[IBIS Ver]   3.2
[File Name]   sprm296a.ibs
[File Rev]   1.0
[Date]   November 3, 2003
[Source]   File originated at Texas Instruments
[Copyright]   (c) 2003, Texas Instruments Inc.
[Component]   f2810pbk
[Manufacturer] Texas Instruments
[Package]
| Variable   Typ   Min   Max
R_pkg   0.063   0.061   0.064
L_pkg   2.512e-09   2.373e-10   2.8e-09
C_pkg   0.455e-13   0.4e-13   0.557e-13
[Pin] signal_name   model_name   R_pin   L_pin   C_pin
1   VDDAIO   NC   0.062 2.856e-09 0.429e-13
2   ADCINB0   ioh125   0.062 2.768e-09 0.518e-13
3   ADCINB1   ioh125   0.061 2.741e-09 0.555e-13
4   ADCINB2   ioh125   0.062 2.718e-09 0.542e-13
5   ADCINB3   ioh125   0.061 2.661e-09 0.499e-13
6   ADCINB4   ioh125   0.061 2.656e-09 0.526e-13
7   ADCINB5   ioh125   0.061 2.604e-09 0.498e-13
8   ADCINB6   ioh125   0.060 2.557e-09 0.432e-13
9   ADCINB7   ioh125   0.061 2.536e-09 0.437e-13
10   ADCREFM   ioh125   0.063 2.528e-09 0.411e-13
11   ADCREFP   ioh125   0.063 2.503e-09 0.376e-13
12   AVSSREFBG   ioh125   0.063 2.456e-09 0.366e-13
13   AVDDREFBG   ioh125   0.064 2.457e-09 0.374e-13
14   VDDA1   NC   0.065 2.457e-09 0.365e-13
15   VSSA1   NC   0.065 2.384e-09 0.330e-13
16   ADCRESEXT   ioh125   0.065 2.337e-09 0.356e-13
17   VSS   NC   0.065 2.341e-09 0.356e-13
18   MDRA   idg095_ouo435_ps1005   0.065 2.380e-09 0.329e-13
19   MDXA   idg095_ouo435   0.065 2.466e-09 0.366e-13
20   VDD   NC   0.065 2.481e-09 0.376e-13
21   MCLKRA   idg095_ouo435_ps1005   0.064 2.479e-09 0.368e-13
22   MFSXA   idg095_ouo435_ps1005   0.063 2.500e-09 0.376e-13
23   MCLKXA   idg095_ouo435_ps1005   0.063 2.528e-09 0.412e-13
24   MFSRA   idg095_ouo435_ps1005   0.062 2.551e-09 0.439e-13
25   VDDIO   NC   0.062 2.591e-09 0.435e-13
26   VSS   NC   0.062 2.636e-09 0.502e-13
27   SPICLKA   idg095_ouo435   0.062 2.663e-09 0.526e-13
28   SPISTEA   idg095_ouo435   0.062 2.676e-09 0.500e-13
29   VDD   NC   0.062 2.731e-09 0.543e-13
30   VSS   NC   0.062 2.763e-09 0.557e-13
31   SPISIMOA   idg095_ouo435   0.063 2.792e-09 0.520e-13
32   SPISOMIA   idg095_ouo435   0.064 2.889e-09 0.432e-13
33   PWM7   sw0145_ouo435_ups285   0.062 2.856e-09 0.429e-13
34   PWM8   sw0145_ouo435_ups285   0.062 2.768e-09 0.518e-13
35   PWM9   sw0145_ouo435_ups285   0.061 2.741e-09 0.555e-13
36   PWM10   sw0145_ouo435_ups285   0.062 2.718e-09 0.542e-13
37   PWM11   sw0145_ouo435_ups285   0.061 2.661e-09 0.499e-13
38   PWM12   sw0145_ouo435_ups285   0.061 2.656e-09 0.526e-13
39   VSS   NC   0.061 2.604e-09 0.498e-13
40   T3PWM_T3CMP   sw0145_ouo435_ups285   0.060 2.557e-09 0.432e-13
41   T4PWM_T4CMP   sw0145_ouo435_ups285   0.061 2.536e-09 0.437e-13
42   VDD   NC   0.063 2.528e-09 0.411e-13
43   CAP4_QEP3   sw0145_ouo435_ups285   0.063 2.503e-09 0.376e-13
44   CAP5_QEP4   sw0145_ouo435_ups285   0.063 2.456e-09 0.366e-13
45   CAP6_QEPI2   sw0145_ouo435_ups285   0.064 2.457e-09 0.374e-13
46   C4TRIPn   sw0145_ouo435_ups285   0.065 2.457e-09 0.365e-13
47   C5TRIPn   sw0145_ouo435_ups285   0.065 2.384e-09 0.330e-13
48   C6TRIPn   sw0145_ouo435_ups285   0.065 2.337e-09 0.356e-13
49   VDDIO   NC   0.065 2.341e-09 0.356e-13
50   TEST2   iog195   0.065 2.380e-09 0.329e-13
51   TEST1   iog195   0.065 2.466e-09 0.366e-13
52   VDD3VFL   NC   0.065 2.481e-09 0.376e-13
53   VSS   NC   0.064 2.479e-09 0.368e-13
54   TDIRB   sw0145_ouo435_ups285   0.063 2.500e-09 0.376e-13
55   TCLKINB   sw0145_ouo435_ups285   0.063 2.528e-09 0.412e-13
56   VDD   NC   0.062 2.551e-09 0.439e-13
57   X2   NC   0.062 2.591e-09 0.435e-13
58   X1/XCLKIN   NC   0.062 2.636e-09 0.502e-13
59   VSS   NC   0.062 2.663e-09 0.526e-13
60   T3CTRIP_PDPINTBn idg095_ouo435_ps1005   0.062 2.676e-09 0.500e-13
61   T4CTRIPn/EVBSOCn idg095_ouo435_ps1005   0.062 2.731e-09 0.543e-13
62   VSS   NC   0.062 2.763e-09 0.557e-13
63   VDD   NC   0.063 2.792e-09 0.520e-13
64	  CANTXA   idg095_ouo435_ps1005 		0.064 2.889e-09 0.43205e-
65	  CANRXA   idg095_ouo435_ps1005 		0.062 2.856e-09 0.42905e-
66	  SCITXDB	  idg095_ouo435   0.062 2.768e-09 0.518e-13
67	  SCIRXDB	  idg095_ouo435   0.061 2.741e-09 0.555e-13
68 	 PWM1	  idg095_ouo435_ps1005   0.062 2.718e-09 0.542e-13
69 	 PWM2   idg095_ouo435_ps1005   0.061 2.661e-09 0.499e-13
70 	 PWM3   idg095_ouo435_ps1005   0.061 2.656e-09 0.526e-13
71	  PWM4   idg095_ouo435_ps1005   0.061 2.604e-09 0.498e-13
72	  PWM5   idg095_ouo435_ps1005   0.060 2.557e-09 0.432e-13
73	  VSS   NC   0.061 2.536e-09 0.437e-13
74	  VDD   NC   0.063 2.528e-09 0.411e-13
75	  PWM6   idg095_ouo435_ps1005   0.063 2.503e-09 0.376e-13
76	 T1PWM_T1CMP	  idg095_ouo435_ps1005   0.063 2.456e-09 0.366e-13
77	  T2PWM_T2CMP	  idg095_ouo435_ps1005   0.064 2.457e-09 0.374e-13
78	 CAP1_QEP1	  idg095_ouo435_ps1005   0.065 2.457e-09 0.365e-13
79	 CAP2_QEP2	  idg095_ouo435_ps1005   0.065 2.384e-09 0.330e-13
80	 CAP3_QEPI1	  idg095_ouo435_ps1005   0.065 2.337e-09 0.356e-13
81	 T1CTRIP_PDPINTAn idg095_ouo435_ps1005   0.065 2.341e-09 0.356e-13
82	 VDD   NC   0.065 2.380e-09 0.329e-13
83 	VDDIO   NC   0.065 2.466e-09 0.366e-13
84	 T2CTRIPn/EVASOCn idg095_ouo435_ps1005   0.065 2.481e-09 0.376e-13
85	 TDIRA   idg095_ouo435_ps1005   0.064 2.479e-09 0.368e-13
86	 TCLKINA	  idg095_ouo435_ps1005   0.063 2.500e-09 0.376e-13
87	 XCLKOUT	  oui835   0.063 2.528e-09 0.412e-13
88	 VSS   NC   0.062 2.551e-09 0.439e-13
89	 C1TRIPn	  idg095_ouo435_ps1005   0.062 2.591e-09 0.435e-13
90	 C2TRIPn	  idg095_ouo435_ps1005   0.062 2.636e-09 0.502e-13
91	 C3TRIPn	  idg095_ouo435_ps1005   0.062 2.663e-09 0.526e-13
92	 TMS   idg095_ps1005   0.062 2.676e-09 0.500e-13
93	 TDO   oui835   0.062 2.731e-09 0.543e-13
94	 VDD   NC   0.062 2.763e-09 0.557e-13
95	 VSS   NC   0.063 2.792e-09 0.520e-13
96	 TDI   idg095_ps1005   0.064 2.889e-09 0.432e-13
97	 TESTSEL	  idg095_pe1005   0.062 2.856e-09 0.429e-13
98	 TRSTn   idg095_pe1005   0.062 2.768e-09 0.518e-13
99	 TCK   idg095_ps1005   0.061 2.741e-09 0.555e-13
100	 EMU0   idg095_oui835_ps1005   0.062 2.718e-09 0.542e-13
101	 XF_XPLLDIS	  idg095_oui835_ps1005   0.061 2.661e-09 0.499e-13
102	 VDD   NC   0.061 2.656e-09 0.526e-13
103	 VSS   NC   0.061 2.604e-09 0.498e-13
104   VDDIO   NC   0.060 2.557e-09 0.432e-13
105   EMU1   idg095_oui835_ps1005 		0.061 2.536e-09 0.437e-13
106   XINT1_XBIOn   idg095_ouo435   0.063 2.528e-09 0.411e-13
107   XNMI_XINT13   idg095_ouo435_ps1005 		0.063 2.503e-09 0.376e-13
108   XINT2_ADCSOC   idg095_ouo435   0.063 2.456e-09 0.366e-13
109   VSS   NC   0.064 2.457e-09 0.374e-13
110   VDD   NC   0.065 2.457e-09 0.365e-13
111   SCITXDA   idg095_ouo435_ps1005 		0.065 2.384e-09 0.330e-13
112   SCIRXDA   idg095_ouo435_ps1005 		0.065 2.337e-09 0.356e-13
113   XRSn   idg095_oum425_ps1005   0.065 2.341e-09 0.356e-13
114   VDD1   NC   0.065 2.380e-09 0.329e-13
115	  VSS1   NC   0.065 2.466e-09 0.366e-13
116   ADCBGREFIN   ioh125   0.065 2.481e-09 0.376e-13
117   VSSA2   NC   0.064 2.479e-09 0.368e-13
118   VDDA2   NC   0.063 2.500e-09 0.376e-13
119   ADCINA7   ioh125   0.063 2.528e-09 0.412e-13
120   ADCINA6   ioh125   0.062 2.551e-09 0.439e-13
121   ADCINA5   ioh125   0.062 2.591e-09 0.435e-13
122   ADCINA4   ioh125   0.062 2.636e-09 0.502e-13
123   ADCINA3   ioh125   0.062 2.663e-09 0.526e-13
124   ADCINA2   ioh125   0.062 2.676e-09 0.500e-13
125   ADCINA1   ioh125   0.062 2.731e-09 0.543e-13
126   ADCINA0   ioh125   0.062 2.763e-09 0.557e-13
127   ADCLO   ioh125   0.063 2.792e-09 0.520e-13
128   VSSAIO   NC   0.064 2.889e-09 0.432e-13
| End of package information
| Component idg095
[Component]   idg095
[Manufacturer]   Texas Instruments
[Package]
|   typ   min   max
R_pkg   0   0   0
L_pkg   0   0   0
C_pkg   0   0   0
[Pin]   signal_name   model_name   R_pin   L_pin   C_pin
   1   A   idg095   0   0   0
| Component idg095_oui835_ps1005
[Component]   idg095_oui835_ps1005
[Manufacturer]   Texas Instruments
[Package]
|   typ   min   max
R_pkg   0   0   0
L_pkg   0   0   0
C_pkg   0   0   0
[Pin]   signal_name   model_name   R_pin   L_pin   C_pin
   1   Y  idg095_oui835_ps1005   0   0   0
| Component idg095_oum425_ps1005
[Component]   idg095_oum425_ps1005
[Manufacturer]   Texas Instruments
[Package]
|   typ   min   max
R_pkg   0   0   0
L_pkg   0   0   0
C_pkg   0   0   0
[Pin]   signal_name   model_name   R_pin   L_pin   C_pin
   1   Y  idg095_oum425_ps1005   0   0   0
| Component idg095_ouo435_ps1005
[Component]   idg095_ouo435_ps1005
[Manufacturer]   Texas Instruments
[Package]
|   typ   min   max
R_pkg   0   0   0
L_pkg   0   0   0
C_pkg   0   0   0
[Pin]   signal_name   model_name   R_pin   L_pin   C_pin
   1   Y  idg095_ouo435_ps1005   0   0   0
| Component idg095_pe1005
[Component]   idg095_pe1005
[Manufacturer]   Texas Instruments
[Package]
|   typ   min   max
R_pkg   0   0   0
L_pkg   0   0   0
C_pkg   0   0   0
[Pin]   signal_name   model_name   R_pin   L_pin   C_pin
   1   A   idg095_pe1005   0   0   0
| Component idg095_ps1005
[Component]   idg095_ps1005
[Manufacturer]   Texas Instruments
[Package]
|   typ   min   max
R_pkg   0   0   0
L_pkg   0   0   0
C_pkg   0   0   0
[Pin]   signal_name   model_name   R_pin   L_pin   C_pin
   1   A   idg095_ps1005   0   0   0
| Component iog195
[Component]   iog195
[Manufacturer]   Texas Instruments
[Package]
|   typ   min   max
R_pkg   0   0   0
L_pkg   0   0   0
C_pkg   0   0   0
[Pin]   signal_name   model_name   R_pin   L_pin   C_pin
   1   Y   iog195   0   0   0
| Component ioh125
[Component]   ioh125
[Manufacturer]   Texas Instruments
[Package]
|   typ   min   max
R_pkg   0   0   0
L_pkg   0   0   0
C_pkg   0   0   0
[Pin]   signal_name   model_name   R_pin   L_pin   C_pin
   1   Y   ioh125   0   0   0
| Component oui835
[Component]   oui835
[Manufacturer]   Texas Instruments
[Package]
|   typ   min   max
R_pkg   0   0   0
L_pkg   0   0   0
C_pkg   0   0   0
[Pin]   signal_name   model_name   R_pin   L_pin   C_pin
   1   Y   oui835   0   0   0
| Component oum425
[Component]   oum425
[Manufacturer]   Texas Instruments
[Package]
|   typ   min   max
R_pkg   0   0   0
L_pkg   0   0   0
C_pkg   0   0   0
[Pin]   signal_name   model_name   R_pin   L_pin   C_pin
   1   Y   oum425   0   0   0
| Component idg095_ouo435
[Component]   idg095_ouo435
[Manufacturer]   Texas Instruments
[Package]
|   typ   min   max
R_pkg   0   0   0
L_pkg   0   0   0
C_pkg   0   0   0
[Pin]   signal_name   model_name   R_pin   L_pin   C_pin
   1   Y   idg095_ouo435   0   0   0
| Component ouo435
[Component]   ouo435
[Manufacturer]   Texas Instruments
[Package]
|   typ   min   max
R_pkg   0   0   0
L_pkg   0   0   0
C_pkg   0   0   0
[Pin]   signal_name   model_name   R_pin   L_pin   C_pin
   1   Y   ouo435   0   0   0
| Component sw0145_ouo435_ups285
[Component]   sw0145_ouo435_ups285
[Manufacturer]   Texas Instruments
[Package]
|   typ   min   max
R_pkg   0   0   0
L_pkg   0   0   0
C_pkg   0   0   0
[Pin]   signal_name   model_name   R_pin   L_pin   C_pin
   1   Y  sw0145_ouo435_ups285   0   0   0
| Models and submodels in the file (13): idg095 (Input), idg095_oui835_ps1005 (I/O), idg095_oum425_ps1005 (I/O_open_sink), idg095_ouo435_ps1005 (I/O), idg095_pe1005 (Input), idg095_ps1005 (Input), iog195 (Terminator), ioh125 (Terminator), oui835 (3-state), oum425 (I/O_open_sink), idg095_ouo435 (I/O), ouo435 (3-state), sw0145_ouo435_ups285 (I/O)
